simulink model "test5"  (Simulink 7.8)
settings: Solver=ode4  StartTime=0.0  StopTime=10.0  FixedStep=1e-2  RelTol=1e-3
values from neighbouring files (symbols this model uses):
  A1 = [0 1; -10 -11]    [ex3_4_parameter.m]
  A2 = [0 1; -10 -2]    [ex3_4_parameter.m]
  A3 = [0 1; -10 0]    [ex3_4_parameter.m]
  B = [0; 1]    [ex3_4_parameter.m]
  C = [1 0]    [ex3_4_parameter.m]
  x0 = [1; 0]    [ex3_4_parameter.m]

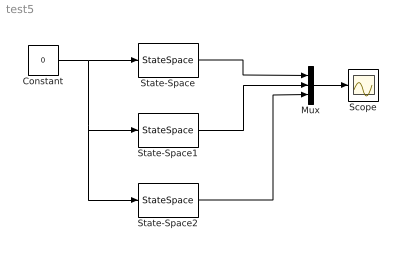
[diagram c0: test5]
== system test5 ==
  Constant : Constant  Value=0
  Mux : Mux  Inputs=3
  Scope : Scope
  State-Space : StateSpace  A=A1  B=B  C=C  D=0  X0=x0
  State-Space1 : StateSpace  A=A2  B=B  C=C  D=0  X0=x0
  State-Space2 : StateSpace  A=A3  B=B  C=C  D=0  X0=x0
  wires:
  Constant/1 -> State-Space/1, State-Space1/1, State-Space2/1
  State-Space/1 -> Mux/1
  State-Space1/1 -> Mux/2
  State-Space2/1 -> Mux/3
  Mux/1 -> Scope/1
